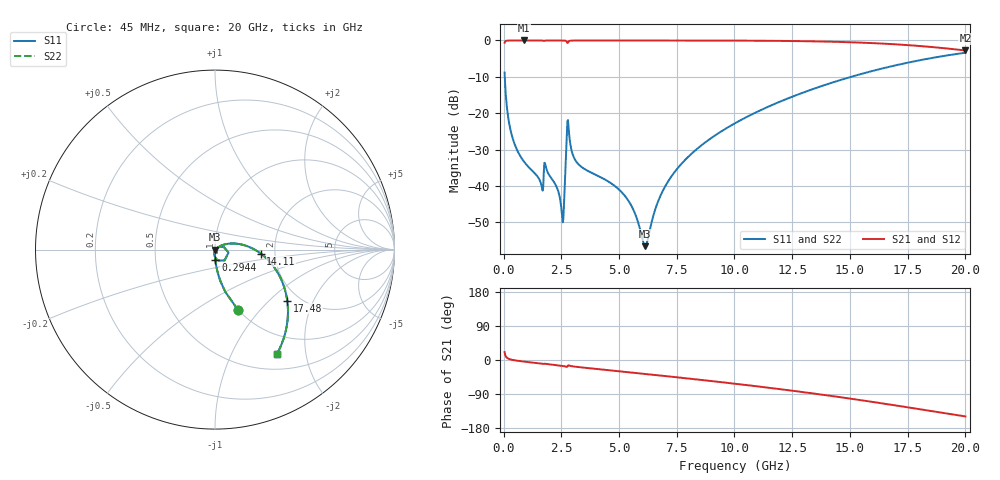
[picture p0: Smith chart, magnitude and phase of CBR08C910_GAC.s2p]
! S-parameter model data by Modelithics Inc.  support@modelithics.com 813-866-6335  Tampa FL USA
! S-Parameter data specifications:
! Substrate: 20-mil Rogers 4350B, substrate thickness, H=0.508mm, Dielectric constant, Er=3.75
! PCB Mounting Pad Footprint: Pad width, PadW=1.45mm , Pad length, PadL=1mm , Pad gap, PadG (edge-to-edge)=0.6mm , Reference planes=2.6mm apart
#  GHz  S  MA  R 50
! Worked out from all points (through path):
!   801 points, 45 MHz to 20 GHz, reference 50 ohm
!   highest |S21| = -0.01 dB at 893.1 MHz (marker M1); lowest = -2.8 dB at 20 GHz (marker M2)
!   group delay of S21, straight-line fit = 20.6 ps
!   lowest |S11| = -56.6 dB at 6.131 GHz (marker M3), VSWR 1.00, Z = 50.1 - j0.0927 ohm
!   |S11| at or under -10 dB: 53.31 MHz to 15.06 GHz (15 GHz wide, 199 % of centre)
!   |S22| runs from -56.6 to -3.4 dB; largest |S21 - S12| = 0
!   S11 on the Smith chart (normalised r, x): 45 MHz: 1.00, -0.77; 294.4 MHz: 1.00, -0.12; 14.11 GHz: 1.68, -0.08; 17.48 GHz: 1.73, -1.30; 20 GHz: 0.70, -1.52
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0.045  0.3614 -69.0  0.932 20.9  0.932 20.9  0.3614 -69.0
0.294438  0.05981 -88.0  0.9978 1.6  0.9978 1.6  0.05981 -88.0
0.893088  0.02138 -92.7  0.9991 -4.3  0.9991 -4.3  0.02138 -92.7
1.616456  0.01083 -91.2  0.9982 -9.3  0.9982 -9.3  0.01083 -91.2
1.865894  0.01666 -92.2  0.9972 -10.5  0.9972 -10.5  0.01666 -92.2
2.314881  0.009399 -95.5  0.9984 -13.6  0.9984 -13.6  0.009399 -95.5
2.514431  0.004499 -75.9  0.9975 -15.1  0.9975 -15.1  0.004499 -75.9
2.589262  0.003535 -6.3  0.9962 -15.8  0.9962 -15.8  0.003535 -6.3
2.738925  0.05129 15.8  0.9568 -18.4  0.9568 -18.4  0.05129 15.8
2.813756  0.06458 -71.6  0.9635 -14.0  0.9635 -14.0  0.06458 -71.6
3.03825  0.02489 -101.2  0.9968 -17.1  0.9968 -17.1  0.02489 -101.2
3.387462  0.01809 -105.1  0.998 -19.6  0.998 -19.6  0.01809 -105.1
5.2333  0.007423 -110.6  0.998 -31.2  0.998 -31.2  0.007423 -110.6
6.131275  0.001482 -38.6  0.9978 -36.8  0.9978 -36.8  0.001482 -38.6
6.704981  0.00627 35.1  0.9977 -40.4  0.9977 -40.4  0.00627 35.1
7.902281  0.02344 37.4  0.9971 -48.2  0.9971 -48.2  0.02344 37.4
10.0225  0.07266 25.6  0.994 -62.6  0.994 -62.6  0.07266 25.6
13.36496  0.2127 1.2  0.9725 -87.9  0.9725 -87.9  0.2127 1.2
14.11327  0.2559 -4.9  0.9617 -94.1  0.9617 -94.1  0.2559 -4.9
16.68248  0.4323 -27.7  0.8953 -117.1  0.8953 -117.1  0.4323 -27.7
17.48068  0.4927 -35.2  0.8633 -124.7  0.8633 -124.7  0.4927 -35.2
20  0.6772 -59.4  0.7274 -148.9  0.7274 -148.9  0.6772 -59.4
